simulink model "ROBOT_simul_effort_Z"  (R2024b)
settings: Solver=VariableStepAuto  StartTime=0.0  StopTime=5  RelTol=1e-3
undefined symbols (not defined in the file): a, ARRIERE_Defaut_sldprt, avant01_Defaut_sldprt, avant02_Defaut_sldprt, avant03_Defaut_sldprt, avant1_Defaut_sldprt, AXE, BASE_Defaut_sldprt, BIELLE, BIELLE_Defaut_sldprt, BRAS_Defaut_sldprt, bras_Defaut_sldprt, C_Realiste_sldprt, CABLE_Defaut_sldprt, cable_Defaut_sldprt, CACHE_Defaut_sldprt, CARTE, carte_Defaut_sldprt, CARTER, carter, CHC, CODEUR_Defaut_sldprt, cruciforme, cylindrique, deg, Drive, Fichiers, Fichiers_Matlab_sujetA, FIXATION, fixation_Defaut_sldprt, H, HEXAGONALE_Defaut_sldprt, joint_Defaut_sldprt, kg, m, M4, M4_Defaut_sldprt, manette1_Defaut_sldprt, manette2_Defaut_sldprt, MATLAB, Matlab, matlab_Defaut_sldprt, mm, modif, MOTEUR_Defaut_sldprt, N, NEZ_Defaut_sldprt, nom, palier, PARALLELOGRAMME_Defaut_sldprt, petite, plaque, rad, Ressort, Rondelle, ROTOR_Defaut_sldprt, s, SET, simple, socle_Defaut_sldprt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
libraries: sm_lib x463, fl_lib x45, nesl_utility x27, simulink x2
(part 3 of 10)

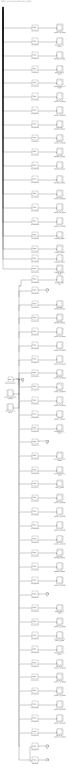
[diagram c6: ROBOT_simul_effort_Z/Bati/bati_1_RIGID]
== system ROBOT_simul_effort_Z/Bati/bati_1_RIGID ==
  CACHE_1_RIGID : Subsystem
  CACHE_2_RIGID : Subsystem
  CACHE_3_RIGID : Subsystem
  CARTER_ARRIERE_1_RIGID : Subsystem
  CARTE_HEXAGONALE_1_RIGID : Subsystem
  FIXATION_MOTEUR_1_RIGID : Subsystem
  FIXATION_MOTEUR_2_RIGID : Subsystem
  FIXATION_MOTEUR_3_RIGID : Subsystem
  FIXATION_MOTEUR_4_RIGID : Subsystem
  FIXATION_MOTEUR_5_RIGID : Subsystem
  FIXATION_MOTEUR_6_RIGID : Subsystem
  MOTEUR_1_RIGID : Subsystem
  MOTEUR_2_RIGID : Subsystem
  MOTEUR_3_RIGID : Subsystem
  PLAQUE_NOM_1_RIGID : Subsystem
  PLAQUE_NOM_SET : Subsystem
  ReferenceFrame : sm_lib/Frames and Transforms/Reference Frame
  Rondelle_M4_1_RIGID : Subsystem
  Rondelle_M4_2_RIGID : Subsystem
  Transform : sm_lib/Frames and Transforms/Rigid Transform  RotationMethod=ArbitraryAxis  FollAlignAxisA=+X  BaseAlignAxisA=+Y  FollAlignAxisB=+Y  BaseAlignAxisB=+Z  RotationStandardAxis=+Z  RotationAngle=2.2576709855630241  RotationAngleUnits=rad  RotationArbitraryAxis=[-0.47317816576134769 -0.62293756647304832 0.62293756647304788]  RotationSequenceAxes=FollowerAxes  RotationSequence=XYX  RotationSequenceAngles=[0 0 0]  RotationSequenceAnglesUnits=deg  RotationMatrix=[1 0 0; 0 1 0; 0 0 1]  Quaternion=[1 0 0 0]  TranslationMethod=Cartesian  TranslationCartesianOffset=[-67.982453021745741 154.13917308955064 38.499999999999979]  TranslationCartesianOffsetUnits=mm  TranslationStandardAxis=+Z  TranslationStandardOffset=0  TranslationStandardOffsetUnits=mm  TranslationROffset=0  TranslationROffsetUnits=m  TranslationThetaOffset=0  TranslationThetaOffsetUnits=deg  TranslationZOffset=0  TranslationZOffsetUnits=m
  Transform1 : sm_lib/Frames and Transforms/Rigid Transform  RotationMethod=ArbitraryAxis  FollAlignAxisA=+X  BaseAlignAxisA=+Y  FollAlignAxisB=+Y  BaseAlignAxisB=+Z  RotationStandardAxis=+Z  RotationAngle=2.2455218567975841  RotationAngleUnits=rad  RotationArbitraryAxis=[-0.62007686508407689 -0.48063433374552811 -0.62007686508407622]  RotationSequenceAxes=FollowerAxes  RotationSequence=XYX  RotationSequenceAngles=[0 0 0]  RotationSequenceAnglesUnits=deg  RotationMatrix=[1 0 0; 0 1 0; 0 0 1]  Quaternion=[1 0 0 0]  TranslationMethod=Cartesian  TranslationCartesianOffset=[67.670238338594061 154.67994478363838 38.499999999999979]  TranslationCartesianOffsetUnits=mm  TranslationStandardAxis=+Z  TranslationStandardOffset=0  TranslationStandardOffsetUnits=mm  TranslationROffset=0  TranslationROffsetUnits=m  TranslationThetaOffset=0  TranslationThetaOffsetUnits=deg  TranslationZOffset=0  TranslationZOffsetUnits=m
  Transform10 : sm_lib/Frames and Transforms/Rigid Transform  RotationMethod=ArbitraryAxis  FollAlignAxisA=+X  BaseAlignAxisA=+Y  FollAlignAxisB=+Y  BaseAlignAxisB=+Z  RotationStandardAxis=+Z  RotationAngle=1.5874169403231204  RotationAngleUnits=rad  RotationArbitraryAxis=[0.12785986324311854 -0.98351599414696989 0.12785986324311688]  RotationSequenceAxes=FollowerAxes  RotationSequence=XYX  RotationSequenceAngles=[0 0 0]  RotationSequenceAnglesUnits=deg  RotationMatrix=[1 0 0; 0 1 0; 0 0 1]  Quaternion=[1 0 0 0]  TranslationMethod=Cartesian  TranslationCartesianOffset=[-21.302011487444762 191.53150356202462 36.100000000000051]  TranslationCartesianOffsetUnits=mm  TranslationStandardAxis=+Z  TranslationStandardOffset=0  TranslationStandardOffsetUnits=mm  TranslationROffset=0  TranslationROffsetUnits=m  TranslationThetaOffset=0  TranslationThetaOffsetUnits=deg  TranslationZOffset=0  TranslationZOffsetUnits=m
  Transform11 : sm_lib/Frames and Transforms/Rigid Transform  RotationMethod=ArbitraryAxis  FollAlignAxisA=+X  BaseAlignAxisA=+Y  FollAlignAxisB=+Y  BaseAlignAxisB=+Z  RotationStandardAxis=+Z  RotationAngle=2.557922199918194  RotationAngleUnits=rad  RotationArbitraryAxis=[0.67444507075713422 -0.30041253812517366 0.67444507075713389]  RotationSequenceAxes=FollowerAxes  RotationSequence=XYX  RotationSequenceAngles=[0 0 0]  RotationSequenceAnglesUnits=deg  RotationMatrix=[1 0 0; 0 1 0; 0 0 1]  Quaternion=[1 0 0 0]  TranslationMethod=Cartesian  TranslationCartesianOffset=[-8.6943864691458312 146.25405010671241 36.099999999999994]  TranslationCartesianOffsetUnits=mm  TranslationStandardAxis=+Z  TranslationStandardOffset=0  TranslationStandardOffsetUnits=mm  TranslationROffset=0  TranslationROffsetUnits=m  TranslationThetaOffset=0  TranslationThetaOffsetUnits=deg  TranslationZOffset=0  TranslationZOffsetUnits=m
  Transform12 : sm_lib/Frames and Transforms/Rigid Transform  RotationMethod=ArbitraryAxis  FollAlignAxisA=+X  BaseAlignAxisA=+Y  FollAlignAxisB=+Y  BaseAlignAxisB=+Z  RotationStandardAxis=+Z  RotationAngle=1.5816892610060764  RotationAngleUnits=rad  RotationArbitraryAxis=[0.10380436397422958 -0.98916596587216399 0.10380436397423064]  RotationSequenceAxes=FollowerAxes  RotationSequence=XYX  RotationSequenceAngles=[0 0 0]  RotationSequenceAnglesUnits=deg  RotationMatrix=[1 0 0; 0 1 0; 0 0 1]  Quaternion=[1 0 0 0]  TranslationMethod=Cartesian  TranslationCartesianOffset=[31.197488247191473 107.27753449924363 36.099999999999994]  TranslationCartesianOffsetUnits=mm  TranslationStandardAxis=+Z  TranslationStandardOffset=0  TranslationStandardOffsetUnits=mm  TranslationROffset=0  TranslationROffsetUnits=m  TranslationThetaOffset=0  TranslationThetaOffsetUnits=deg  TranslationZOffset=0  TranslationZOffsetUnits=m
  Transform13 : sm_lib/Frames and Transforms/Rigid Transform  RotationMethod=ArbitraryAxis  FollAlignAxisA=+X  BaseAlignAxisA=+Y  FollAlignAxisB=+Y  BaseAlignAxisB=+Z  RotationStandardAxis=+Z  RotationAngle=2.4188584057763718  RotationAngleUnits=rad  RotationArbitraryAxis=[-0.65465367070797598 -0.37796447300923064 -0.6546536707079762]  RotationSequenceAxes=FollowerAxes  RotationSequence=XYX  RotationSequenceAngles=[0 0 0]  RotationSequenceAnglesUnits=deg  RotationMatrix=[1 0 0; 0 1 0; 0 0 1]  Quaternion=[1 0 0 0]  TranslationMethod=Cartesian  TranslationCartesianOffset=[-32.1104315373926 141.51053427005223 49.100000000000001]  TranslationCartesianOffsetUnits=mm  TranslationStandardAxis=+Z  TranslationStandardOffset=0  TranslationStandardOffsetUnits=mm  TranslationROffset=0  TranslationROffsetUnits=m  TranslationThetaOffset=0  TranslationThetaOffsetUnits=deg  TranslationZOffset=0  TranslationZOffsetUnits=m
  Transform14 : sm_lib/Frames and Transforms/Rigid Transform  RotationMethod=ArbitraryAxis  FollAlignAxisA=+X  BaseAlignAxisA=+Y  FollAlignAxisB=+Y  BaseAlignAxisB=+Z  RotationStandardAxis=+Z  RotationAngle=2.253606277940353  RotationAngleUnits=rad  RotationArbitraryAxis=[-0.62198874395633519 -0.47566795643940651 -0.62198874395633508]  RotationSequenceAxes=FollowerAxes  RotationSequence=XYX  RotationSequenceAngles=[0 0 0]  RotationSequenceAnglesUnits=deg  RotationMatrix=[1 0 0; 0 1 0; 0 0 1]  Quaternion=[1 0 0 0]  TranslationMethod=Cartesian  TranslationCartesianOffset=[76.71272566730876 95.557331318822435 36.100000000000051]  TranslationCartesianOffsetUnits=mm  TranslationStandardAxis=+Z  TranslationStandardOffset=0  TranslationStandardOffsetUnits=mm  TranslationROffset=0  TranslationROffsetUnits=m  TranslationThetaOffset=0  TranslationThetaOffsetUnits=deg  TranslationZOffset=0  TranslationZOffsetUnits=m
  Transform15 : sm_lib/Frames and Transforms/Rigid Transform  RotationMethod=ArbitraryAxis  FollAlignAxisA=+X  BaseAlignAxisA=+Y  FollAlignAxisB=+Y  BaseAlignAxisB=+Z  RotationStandardAxis=+Z  RotationAngle=2.1395291955010958  RotationAngleUnits=rad  RotationArbitraryAxis=[-0.59164485304725056 -0.54764289069191197 -0.59164485304725156]  RotationSequenceAxes=FollowerAxes  RotationSequence=XYX  RotationSequenceAngles=[0 0 0]  RotationSequenceAnglesUnits=deg  RotationMatrix=[1 0 0; 0 1 0; 0 0 1]  Quaternion=[1 0 0 0]  TranslationMethod=Cartesian  TranslationCartesianOffset=[39.05251803832482 137.78242766379034 36.099999999999966]  TranslationCartesianOffsetUnits=mm  TranslationStandardAxis=+Z  TranslationStandardOffset=0  TranslationStandardOffsetUnits=mm  TranslationROffset=0  TranslationROffsetUnits=m  TranslationThetaOffset=0  TranslationThetaOffsetUnits=deg  TranslationZOffset=0  TranslationZOffsetUnits=m
  Transform16 : sm_lib/Frames and Transforms/Rigid Transform  RotationMethod=ArbitraryAxis  FollAlignAxisA=+X  BaseAlignAxisA=+Y  FollAlignAxisB=+Y  BaseAlignAxisB=+Z  RotationStandardAxis=+Z  RotationAngle=0.1305039651717789  RotationAngleUnits=rad  RotationArbitraryAxis=[1.6038157489539324e-15 1 -1.2797090690177757e-15]  RotationSequenceAxes=FollowerAxes  RotationSequence=XYX  RotationSequenceAngles=[0 0 0]  RotationSequenceAnglesUnits=deg  RotationMatrix=[1 0 0; 0 1 0; 0 0 1]  Quaternion=[1 0 0 0]  TranslationMethod=Cartesian  TranslationCartesianOffset=[-9.8750000000000053 1.2000000000000066 14.050000000000008]  TranslationCartesianOffsetUnits=mm  TranslationStandardAxis=+Z  TranslationStandardOffset=0  TranslationStandardOffsetUnits=mm  TranslationROffset=0  TranslationROffsetUnits=m  TranslationThetaOffset=0  TranslationThetaOffsetUnits=deg  TranslationZOffset=0  TranslationZOffsetUnits=m
  Transform17 : sm_lib/Frames and Transforms/Rigid Transform  RotationMethod=ArbitraryAxis  FollAlignAxisA=+X  BaseAlignAxisA=+Y  FollAlignAxisB=+Y  BaseAlignAxisB=+Z  RotationStandardAxis=+Z  RotationAngle=3.1415926535897931  RotationAngleUnits=rad  RotationArbitraryAxis=[-0.14780941112961105 0.98901586336191671 0]  RotationSequenceAxes=FollowerAxes  RotationSequence=XYX  RotationSequenceAngles=[0 0 0]  RotationSequenceAnglesUnits=deg  RotationMatrix=[1 0 0; 0 1 0; 0 0 1]  Quaternion=[1 0 0 0]  TranslationMethod=Cartesian  TranslationCartesianOffset=[0 115.25000000000001 16.899999999999999]  TranslationCartesianOffsetUnits=mm  TranslationStandardAxis=+Z  TranslationStandardOffset=0  TranslationStandardOffsetUnits=mm  TranslationROffset=0  TranslationROffsetUnits=m  TranslationThetaOffset=0  TranslationThetaOffsetUnits=deg  TranslationZOffset=0  TranslationZOffsetUnits=m
  Transform18 : sm_lib/Frames and Transforms/Rigid Transform  RotationMethod=ArbitraryAxis  FollAlignAxisA=+X  BaseAlignAxisA=+Y  FollAlignAxisB=+Y  BaseAlignAxisB=+Z  RotationStandardAxis=+Z  RotationAngle=3.1415926535897909  RotationAngleUnits=rad  RotationArbitraryAxis=[-0.70710678118654757 -1.2168216554799258e-15 -0.70710678118654746]  RotationSequenceAxes=FollowerAxes  RotationSequence=XYX  RotationSequenceAngles=[0 0 0]  RotationSequenceAnglesUnits=deg  RotationMatrix=[1 0 0; 0 1 0; 0 0 1]  Quaternion=[1 0 0 0]  TranslationMethod=Cartesian  TranslationCartesianOffset=[0 115.25000000000001 -1.799999999999996]  TranslationCartesianOffsetUnits=mm  TranslationStandardAxis=+Z  TranslationStandardOffset=0  TranslationStandardOffsetUnits=mm  TranslationROffset=0  TranslationROffsetUnits=m  TranslationThetaOffset=0  TranslationThetaOffsetUnits=deg  TranslationZOffset=0  TranslationZOffsetUnits=m
  Transform19 : sm_lib/Frames and Transforms/Rigid Transform  RotationMethod=ArbitraryAxis  FollAlignAxisA=+X  BaseAlignAxisA=+Y  FollAlignAxisB=+Y  BaseAlignAxisB=+Z  RotationStandardAxis=+Z  RotationAngle=3.1415926535897931  RotationAngleUnits=rad  RotationArbitraryAxis=[-0.62251463663761875 0.78260815685241447 9.5278235956943858e-17]  RotationSequenceAxes=FollowerAxes  RotationSequence=XYX  RotationSequenceAngles=[0 0 0]  RotationSequenceAnglesUnits=deg  RotationMatrix=[1 0 0; 0 1 0; 0 0 1]  Quaternion=[1 0 0 0]  TranslationMethod=Cartesian  TranslationCartesianOffset=[-5.4923264138695282 106.15877278095202 52.900000000000013]  TranslationCartesianOffsetUnits=mm  TranslationStandardAxis=+Z  TranslationStandardOffset=0  TranslationStandardOffsetUnits=mm  TranslationROffset=0  TranslationROffsetUnits=m  TranslationThetaOffset=0  TranslationThetaOffsetUnits=deg  TranslationZOffset=0  TranslationZOffsetUnits=m
  Transform2 : sm_lib/Frames and Transforms/Rigid Transform  RotationMethod=ArbitraryAxis  FollAlignAxisA=+X  BaseAlignAxisA=+Y  FollAlignAxisB=+Y  BaseAlignAxisB=+Z  RotationStandardAxis=+Z  RotationAngle=1.7212826903554606  RotationAngleUnits=rad  RotationArbitraryAxis=[0.85979818153437826 0.36107276761767659 0.36107276761767548]  RotationSequenceAxes=FollowerAxes  RotationSequence=XYX  RotationSequenceAngles=[0 0 0]  RotationSequenceAnglesUnits=deg  RotationMatrix=[1 0 0; 0 1 0; 0 0 1]  Quaternion=[1 0 0 0]  TranslationMethod=Cartesian  TranslationCartesianOffset=[0.3122146831511497 36.930882126810701 38.499999999999979]  TranslationCartesianOffsetUnits=mm  TranslationStandardAxis=+Z  TranslationStandardOffset=0  TranslationStandardOffsetUnits=mm  TranslationROffset=0  TranslationROffsetUnits=m  TranslationThetaOffset=0  TranslationThetaOffsetUnits=deg  TranslationZOffset=0  TranslationZOffsetUnits=m
  Transform20 : sm_lib/Frames and Transforms/Rigid Transform  RotationMethod=ArbitraryAxis  FollAlignAxisA=+X  BaseAlignAxisA=+Y  FollAlignAxisB=+Y  BaseAlignAxisB=+Z  RotationStandardAxis=+Z  RotationAngle=1.5707963267948968  RotationAngleUnits=rad  RotationArbitraryAxis=[-0 -1 -1.8723979605913744e-16]  RotationSequenceAxes=FollowerAxes  RotationSequence=XYX  RotationSequenceAngles=[0 0 0]  RotationSequenceAnglesUnits=deg  RotationMatrix=[1 0 0; 0 1 0; 0 0 1]  Quaternion=[1 0 0 0]  TranslationMethod=Cartesian  TranslationCartesianOffset=[-6.6870740261211532 74.311283427110965 49.100000000000001]  TranslationCartesianOffsetUnits=mm  TranslationStandardAxis=+Z  TranslationStandardOffset=0  TranslationStandardOffsetUnits=mm  TranslationROffset=0  TranslationROffsetUnits=m  TranslationThetaOffset=0  TranslationThetaOffsetUnits=deg  TranslationZOffset=0  TranslationZOffsetUnits=m
  Transform21 : sm_lib/Frames and Transforms/Rigid Transform  RotationMethod=ArbitraryAxis  FollAlignAxisA=+X  BaseAlignAxisA=+Y  FollAlignAxisB=+Y  BaseAlignAxisB=+Z  RotationStandardAxis=+Z  RotationAngle=2.5869353710023297  RotationAngleUnits=rad  RotationArbitraryAxis=[-0.28466429222446077 0.67785184248932562 -0.6778518424893254]  RotationSequenceAxes=FollowerAxes  RotationSequence=XYX  RotationSequenceAngles=[0 0 0]  RotationSequenceAnglesUnits=deg  RotationMatrix=[1 0 0; 0 1 0; 0 0 1]  Quaternion=[1 0 0 0]  TranslationMethod=Cartesian  TranslationCartesianOffset=[-16.466410454294302 53.38468832772007 38.500000000000007]  TranslationCartesianOffsetUnits=mm  TranslationStandardAxis=+Z  TranslationStandardOffset=0  TranslationStandardOffsetUnits=mm  TranslationROffset=0  TranslationROffsetUnits=m  TranslationThetaOffset=0  TranslationThetaOffsetUnits=deg  TranslationZOffset=0  TranslationZOffsetUnits=m
  Transform22 : sm_lib/Frames and Transforms/Rigid Transform  RotationMethod=ArbitraryAxis  FollAlignAxisA=+X  BaseAlignAxisA=+Y  FollAlignAxisB=+Y  BaseAlignAxisB=+Z  RotationStandardAxis=+Z  RotationAngle=2.5869353710023297  RotationAngleUnits=rad  RotationArbitraryAxis=[-0.28466429222446077 0.67785184248932562 -0.67785184248932528]  RotationSequenceAxes=FollowerAxes  RotationSequence=XYX  RotationSequenceAngles=[0 0 0]  RotationSequenceAnglesUnits=deg  RotationMatrix=[1 0 0; 0 1 0; 0 0 1]  Quaternion=[1 0 0 0]  TranslationMethod=Cartesian  TranslationCartesianOffset=[-38.956907978955229 75.439790256598585 38.500000000000028]  TranslationCartesianOffsetUnits=mm  TranslationStandardAxis=+Z  TranslationStandardOffset=0  TranslationStandardOffsetUnits=mm  TranslationROffset=0  TranslationROffsetUnits=m  TranslationThetaOffset=0  TranslationThetaOffsetUnits=deg  TranslationZOffset=0  TranslationZOffsetUnits=m
  Transform23 : sm_lib/Frames and Transforms/Rigid Transform  RotationMethod=ArbitraryAxis  FollAlignAxisA=+X  BaseAlignAxisA=+Y  FollAlignAxisB=+Y  BaseAlignAxisB=+Z  RotationStandardAxis=+Z  RotationAngle=2.1079572963404796  RotationAngleUnits=rad  RotationArbitraryAxis=[0.58180115951651357 -0.56834392894662011 0.58180115951651357]  RotationSequenceAxes=FollowerAxes  RotationSequence=XYX  RotationSequenceAngles=[0 0 0]  RotationSequenceAnglesUnits=deg  RotationMatrix=[1 0 0; 0 1 0; 0 0 1]  Quaternion=[1 0 0 0]  TranslationMethod=Cartesian  TranslationCartesianOffset=[-32.920216655203667 36.606063190274597 36.100000000000037]  TranslationCartesianOffsetUnits=mm  TranslationStandardAxis=+Z  TranslationStandardOffset=0  TranslationStandardOffsetUnits=mm  TranslationROffset=0  TranslationROffsetUnits=m  TranslationThetaOffset=0  TranslationThetaOffsetUnits=deg  TranslationZOffset=0  TranslationZOffsetUnits=m
  Transform24 : sm_lib/Frames and Transforms/Rigid Transform  RotationMethod=ArbitraryAxis  FollAlignAxisA=+X  BaseAlignAxisA=+Y  FollAlignAxisB=+Y  BaseAlignAxisB=+Z  RotationStandardAxis=+Z  RotationAngle=2.5913633997650876  RotationAngleUnits=rad  RotationArbitraryAxis=[0.67835179231251819 -0.28227237153641171 0.67835179231251697]  RotationSequenceAxes=FollowerAxes  RotationSequence=XYX  RotationSequenceAngles=[0 0 0]  RotationSequenceAnglesUnits=deg  RotationMatrix=[1 0 0; 0 1 0; 0 0 1]  Quaternion=[1 0 0 0]  TranslationMethod=Cartesian  TranslationCartesianOffset=[-55.410714179864605 58.661165119153118 36.100000000000051]  TranslationCartesianOffsetUnits=mm  TranslationStandardAxis=+Z  TranslationStandardOffset=0  TranslationStandardOffsetUnits=mm  TranslationROffset=0  TranslationROffsetUnits=m  TranslationThetaOffset=0  TranslationThetaOffsetUnits=deg  TranslationZOffset=0  TranslationZOffsetUnits=m
  Transform25 : sm_lib/Frames and Transforms/Rigid Transform  RotationMethod=ArbitraryAxis  FollAlignAxisA=+X  BaseAlignAxisA=+Y  FollAlignAxisB=+Y  BaseAlignAxisB=+Z  RotationStandardAxis=+Z  RotationAngle=2.7200049334585095  RotationAngleUnits=rad  RotationArbitraryAxis=[0.6907299635194234 -0.21397250990001554 0.6907299635194234]  RotationSequenceAxes=FollowerAxes  RotationSequence=XYX  RotationSequenceAngles=[0 0 0]  RotationSequenceAnglesUnits=deg  RotationMatrix=[1 0 0; 0 1 0; 0 0 1]  Quaternion=[1 0 0 0]  TranslationMethod=Cartesian  TranslationCartesianOffset=[-0.012604253384927124 70.163313465165515 36.099999999999966]  TranslationCartesianOffsetUnits=mm  TranslationStandardAxis=+Z  TranslationStandardOffset=0  TranslationStandardOffsetUnits=mm  TranslationROffset=0  TranslationROffsetUnits=m  TranslationThetaOffset=0  TranslationThetaOffsetUnits=deg  TranslationZOffset=0  TranslationZOffsetUnits=m
  Transform26 : sm_lib/Frames and Transforms/Rigid Transform  RotationMethod=ArbitraryAxis  FollAlignAxisA=+X  BaseAlignAxisA=+Y  FollAlignAxisB=+Y  BaseAlignAxisB=+Z  RotationStandardAxis=+Z  RotationAngle=2.2845314039372839  RotationAngleUnits=rad  RotationArbitraryAxis=[-0.62900467206978528 -0.4568437862429186 -0.62900467206978417]  RotationSequenceAxes=FollowerAxes  RotationSequence=XYX  RotationSequenceAngles=[0 0 0]  RotationSequenceAnglesUnits=deg  RotationMatrix=[1 0 0; 0 1 0; 0 0 1]  Quaternion=[1 0 0 0]  TranslationMethod=Cartesian  TranslationCartesianOffset=[-22.503101778045874 92.21841539404403 36.099999999999994]  TranslationCartesianOffsetUnits=mm  TranslationStandardAxis=+Z  TranslationStandardOffset=0  TranslationStandardOffsetUnits=mm  TranslationROffset=0  TranslationROffsetUnits=m  TranslationThetaOffset=0  TranslationThetaOffsetUnits=deg  TranslationZOffset=0  TranslationZOffsetUnits=m
  Transform27 : sm_lib/Frames and Transforms/Rigid Transform  RotationMethod=ArbitraryAxis  FollAlignAxisA=+X  BaseAlignAxisA=+Y  FollAlignAxisB=+Y  BaseAlignAxisB=+Z  RotationStandardAxis=+Z  RotationAngle=1.5707963267948961  RotationAngleUnits=rad  RotationArbitraryAxis=[-1 0 0]  RotationSequenceAxes=FollowerAxes  RotationSequence=XYX  RotationSequenceAngles=[0 0 0]  RotationSequenceAnglesUnits=deg  RotationMatrix=[1 0 0; 0 1 0; 0 0 1]  Quaternion=[1 0 0 0]  TranslationMethod=Cartesian  TranslationCartesianOffset=[0 -1.5000000000000151 37.700000000000003]  TranslationCartesianOffsetUnits=mm  TranslationStandardAxis=+Z  TranslationStandardOffset=0  TranslationStandardOffsetUnits=mm  TranslationROffset=0  TranslationROffsetUnits=m  TranslationThetaOffset=0  TranslationThetaOffsetUnits=deg  TranslationZOffset=0  TranslationZOffsetUnits=m
  Transform28 : sm_lib/Frames and Transforms/Rigid Transform  RotationMethod=ArbitraryAxis  FollAlignAxisA=+X  BaseAlignAxisA=+Y  FollAlignAxisB=+Y  BaseAlignAxisB=+Z  RotationStandardAxis=+Z  RotationAngle=2.773492570857111  RotationAngleUnits=rad  RotationArbitraryAxis=[0.18615678789738549 -0.69474659060686594 0.69474659060686572]  RotationSequenceAxes=FollowerAxes  RotationSequence=XYX  RotationSequenceAngles=[0 0 0]  RotationSequenceAnglesUnits=deg  RotationMatrix=[1 0 0; 0 1 0; 0 0 1]  Quaternion=[1 0 0 0]  TranslationMethod=Cartesian  TranslationCartesianOffset=[9.8750000000000089 31.199999999999992 14.050000000000008]  TranslationCartesianOffsetUnits=mm  TranslationStandardAxis=+Z  TranslationStandardOffset=0  TranslationStandardOffsetUnits=mm  TranslationROffset=0  TranslationROffsetUnits=m  TranslationThetaOffset=0  TranslationThetaOffsetUnits=deg  TranslationZOffset=0  TranslationZOffsetUnits=m
  Transform29 : sm_lib/Frames and Transforms/Rigid Transform  RotationMethod=ArbitraryAxis  FollAlignAxisA=+X  BaseAlignAxisA=+Y  FollAlignAxisB=+Y  BaseAlignAxisB=+Z  RotationStandardAxis=+Z  RotationAngle=2.773492570857111  RotationAngleUnits=rad  RotationArbitraryAxis=[0.18615678789738549 -0.69474659060686594 0.69474659060686572]  RotationSequenceAxes=FollowerAxes  RotationSequence=XYX  RotationSequenceAngles=[0 0 0]  RotationSequenceAnglesUnits=deg  RotationMatrix=[1 0 0; 0 1 0; 0 0 1]  Quaternion=[1 0 0 0]  TranslationMethod=Cartesian  TranslationCartesianOffset=[-9.8750000000000053 31.199999999999992 14.050000000000008]  TranslationCartesianOffsetUnits=mm  TranslationStandardAxis=+Z  TranslationStandardOffset=0  TranslationStandardOffsetUnits=mm  TranslationROffset=0  TranslationROffsetUnits=m  TranslationThetaOffset=0  TranslationThetaOffsetUnits=deg  TranslationZOffset=0  TranslationZOffsetUnits=m
  Transform3 : sm_lib/Frames and Transforms/Rigid Transform  RotationMethod=ArbitraryAxis  FollAlignAxisA=+X  BaseAlignAxisA=+Y  FollAlignAxisB=+Y  BaseAlignAxisB=+Z  RotationStandardAxis=+Z  RotationAngle=1.7212826903554632  RotationAngleUnits=rad  RotationArbitraryAxis=[0.85979818153438259 0.36107276761767909 0.36107276761766205]  RotationSequenceAxes=FollowerAxes  RotationSequence=XYX  RotationSequenceAngles=[0 0 0]  RotationSequenceAnglesUnits=deg  RotationMatrix=[1 0 0; 0 1 0; 0 0 1]  Quaternion=[1 0 0 0]  TranslationMethod=Cartesian  TranslationCartesianOffset=[-106.82639785458468 167.86430788780581 99.318100970001225]  TranslationCartesianOffsetUnits=mm  TranslationStandardAxis=+Z  TranslationStandardOffset=0  TranslationStandardOffsetUnits=mm  TranslationROffset=0  TranslationROffsetUnits=m  TranslationThetaOffset=0  TranslationThetaOffsetUnits=deg  TranslationZOffset=0  TranslationZOffsetUnits=m
  Transform30 : sm_lib/Frames and Transforms/Rigid Transform  RotationMethod=ArbitraryAxis  FollAlignAxisA=+X  BaseAlignAxisA=+Y  FollAlignAxisB=+Y  BaseAlignAxisB=+Z  RotationStandardAxis=+Z  RotationAngle=3.1415926535897931  RotationAngleUnits=rad  RotationArbitraryAxis=[-0.99787184465383982 -0 0.065205687230048659]  RotationSequenceAxes=FollowerAxes  RotationSequence=XYX  RotationSequenceAngles=[0 0 0]  RotationSequenceAnglesUnits=deg  RotationMatrix=[1 0 0; 0 1 0; 0 0 1]  Quaternion=[1 0 0 0]  TranslationMethod=Cartesian  TranslationCartesianOffset=[9.8750000000000089 2.0000000000000018 14.050000000000008]  TranslationCartesianOffsetUnits=mm  TranslationStandardAxis=+Z  TranslationStandardOffset=0  TranslationStandardOffsetUnits=mm  TranslationROffset=0  TranslationROffsetUnits=m  TranslationThetaOffset=0  TranslationThetaOffsetUnits=deg  TranslationZOffset=0  TranslationZOffsetUnits=m
  Transform31 : sm_lib/Frames and Transforms/Rigid Transform  RotationMethod=ArbitraryAxis  FollAlignAxisA=+X  BaseAlignAxisA=+Y  FollAlignAxisB=+Y  BaseAlignAxisB=+Z  RotationStandardAxis=+Z  RotationAngle=3.1415926535897931  RotationAngleUnits=rad  RotationArbitraryAxis=[0 1 0]  RotationSequenceAxes=FollowerAxes  RotationSequence=XYX  RotationSequenceAngles=[0 0 0]  RotationSequenceAnglesUnits=deg  RotationMatrix=[1 0 0; 0 1 0; 0 0 1]  Quaternion=[1 0 0 0]  TranslationMethod=None  TranslationCartesianOffset=[0 0 0]  TranslationCartesianOffsetUnits=m  TranslationStandardAxis=+Z  TranslationStandardOffset=0  TranslationStandardOffsetUnits=m  TranslationROffset=0  TranslationROffsetUnits=m  TranslationThetaOffset=0  TranslationThetaOffsetUnits=deg  TranslationZOffset=0  TranslationZOffsetUnits=m
  Transform32 : sm_lib/Frames and Transforms/Rigid Transform  RotationMethod=ArbitraryAxis  FollAlignAxisA=+X  BaseAlignAxisA=+Y  FollAlignAxisB=+Y  BaseAlignAxisB=+Z  RotationStandardAxis=+Z  RotationAngle=1.6591931073504684  RotationAngleUnits=rad  RotationArbitraryAxis=[-0.28481620059537222 -0.91529201010214944 -0.28481620059537222]  RotationSequenceAxes=FollowerAxes  RotationSequence=XYX  RotationSequenceAngles=[0 0 0]  RotationSequenceAnglesUnits=deg  RotationMatrix=[1 0 0; 0 1 0; 0 0 1]  Quaternion=[1 0 0 0]  TranslationMethod=Cartesian  TranslationCartesianOffset=[78.177113545509911 88.894999319852587 19.199999999999996]  TranslationCartesianOffsetUnits=mm  TranslationStandardAxis=+Z  TranslationStandardOffset=0  TranslationStandardOffsetUnits=mm  TranslationROffset=0  TranslationROffsetUnits=m  TranslationThetaOffset=0  TranslationThetaOffsetUnits=deg  TranslationZOffset=0  TranslationZOffsetUnits=m
  Transform33 : sm_lib/Frames and Transforms/Rigid Transform  RotationMethod=ArbitraryAxis  FollAlignAxisA=+X  BaseAlignAxisA=+Y  FollAlignAxisB=+Y  BaseAlignAxisB=+Z  RotationStandardAxis=+Z  RotationAngle=1.5707963267948968  RotationAngleUnits=rad  RotationArbitraryAxis=[-0 -1 -0]  RotationSequenceAxes=FollowerAxes  RotationSequence=XYX  RotationSequenceAngles=[0 0 0]  RotationSequenceAnglesUnits=deg  RotationMatrix=[1 0 0; 0 1 0; 0 0 1]  Quaternion=[1 0 0 0]  TranslationMethod=Cartesian  TranslationCartesianOffset=[56.590549141302901 55.218676943733961 19.199999999999996]  TranslationCartesianOffsetUnits=mm  TranslationStandardAxis=+Z  TranslationStandardOffset=0  TranslationStandardOffsetUnits=mm  TranslationROffset=0  TranslationROffsetUnits=m  TranslationThetaOffset=0  TranslationThetaOffsetUnits=deg  TranslationZOffset=0  TranslationZOffsetUnits=m
  Transform34 : sm_lib/Frames and Transforms/Rigid Transform  RotationMethod=ArbitraryAxis  FollAlignAxisA=+X  BaseAlignAxisA=+Y  FollAlignAxisB=+Y  BaseAlignAxisB=+Z  RotationStandardAxis=+Z  RotationAngle=2.4188584057763807  RotationAngleUnits=rad  RotationArbitraryAxis=[0.65465367070797764 -0.37796447300922553 0.65465367070797764]  RotationSequenceAxes=FollowerAxes  RotationSequence=XYX  RotationSequenceAngles=[0 0 0]  RotationSequenceAnglesUnits=deg  RotationMatrix=[1 0 0; 0 1 0; 0 0 1]  Quaternion=[1 0 0 0]  TranslationMethod=Cartesian  TranslationCartesianOffset=[23.693376218865065 194.27451469861313 19.199999999999996]  TranslationCartesianOffsetUnits=mm  TranslationStandardAxis=+Z  TranslationStandardOffset=0  TranslationStandardOffsetUnits=mm  TranslationROffset=0  TranslationROffsetUnits=m  TranslationThetaOffset=0  TranslationThetaOffsetUnits=deg  TranslationZOffset=0  TranslationZOffsetUnits=m
  Transform35 : sm_lib/Frames and Transforms/Rigid Transform  RotationMethod=ArbitraryAxis  FollAlignAxisA=+X  BaseAlignAxisA=+Y  FollAlignAxisB=+Y  BaseAlignAxisB=+Z  RotationStandardAxis=+Z  RotationAngle=2.4188584057763718  RotationAngleUnits=rad  RotationArbitraryAxis=[-0.65465367070797598 -0.37796447300923064 -0.65465367070797609]  RotationSequenceAxes=FollowerAxes  RotationSequence=XYX  RotationSequenceAngles=[0 0 0]  RotationSequenceAnglesUnits=deg  RotationMatrix=[1 0 0; 0 1 0; 0 0 1]  Quaternion=[1 0 0 0]  TranslationMethod=Cartesian  TranslationCartesianOffset=[-80.283925360168155 96.256808357652318 19.199999999999996]  TranslationCartesianOffsetUnits=mm  TranslationStandardAxis=+Z  TranslationStandardOffset=0  TranslationStandardOffsetUnits=mm  TranslationROffset=0  TranslationROffsetUnits=m  TranslationThetaOffset=0  TranslationThetaOffsetUnits=deg  TranslationZOffset=0  TranslationZOffsetUnits=m
  Transform36 : sm_lib/Frames and Transforms/Rigid Transform  RotationMethod=ArbitraryAxis  FollAlignAxisA=+X  BaseAlignAxisA=+Y  FollAlignAxisB=+Y  BaseAlignAxisB=+Z  RotationStandardAxis=+Z  RotationAngle=2.0489764020053052  RotationAngleUnits=rad  RotationArbitraryAxis=[0.56137820698022478 -0.60803701980663627 0.56137820698022478]  RotationSequenceAxes=FollowerAxes  RotationSequence=XYX  RotationSequenceAngles=[0 0 0]  RotationSequenceAnglesUnits=deg  RotationMatrix=[1 0 0; 0 1 0; 0 0 1]  Quaternion=[1 0 0 0]  TranslationMethod=Cartesian  TranslationCartesianOffset=[-16.264456666991514 196.13086666502576 19.199999999999996]  TranslationCartesianOffsetUnits=mm  TranslationStandardAxis=+Z  TranslationStandardOffset=0  TranslationStandardOffsetUnits=mm  TranslationROffset=0  TranslationROffsetUnits=m  TranslationThetaOffset=0  TranslationThetaOffsetUnits=deg  TranslationZOffset=0  TranslationZOffsetUnits=m
  Transform37 : sm_lib/Frames and Transforms/Rigid Transform  RotationMethod=ArbitraryAxis  FollAlignAxisA=+X  BaseAlignAxisA=+Y  FollAlignAxisB=+Y  BaseAlignAxisB=+Z  RotationStandardAxis=+Z  RotationAngle=2.8290477720117608  RotationAngleUnits=rad  RotationArbitraryAxis=[-0.69827493103712956 -0.15755710510854135 -0.69827493103712956]  RotationSequenceAxes=FollowerAxes  RotationSequence=XYX  RotationSequenceAngles=[0 0 0]  RotationSequenceAnglesUnits=deg  RotationMatrix=[1 0 0; 0 1 0; 0 0 1]  Quaternion=[1 0 0 0]  TranslationMethod=Cartesian  TranslationCartesianOffset=[-61.912656878518263 60.724134015121031 19.199999999999996]  TranslationCartesianOffsetUnits=mm  TranslationStandardAxis=+Z  TranslationStandardOffset=0  TranslationStandardOffsetUnits=mm  TranslationROffset=0  TranslationROffsetUnits=m  TranslationThetaOffset=0  TranslationThetaOffsetUnits=deg  TranslationZOffset=0  TranslationZOffsetUnits=m
  Transform38 : sm_lib/Frames and Transforms/Rigid Transform  RotationMethod=ArbitraryAxis  FollAlignAxisA=+X  BaseAlignAxisA=+Y  FollAlignAxisB=+Y  BaseAlignAxisB=+Z  RotationStandardAxis=+Z  RotationAngle=1.5865923302678127  RotationAngleUnits=rad  RotationArbitraryAxis=[-0.98432745245712761 0.12469856923650155 -0.1246985692365027]  RotationSequenceAxes=FollowerAxes  RotationSequence=XYX  RotationSequenceAngles=[0 0 0]  RotationSequenceAnglesUnits=deg  RotationMatrix=[1 0 0; 0 1 0; 0 0 1]  Quaternion=[1 0 0 0]  TranslationMethod=Cartesian  TranslationCartesianOffset=[61.810136748383464 131.92232607357974 38.500000000000007]  TranslationCartesianOffsetUnits=mm  TranslationStandardAxis=+Z  TranslationStandardOffset=0  TranslationStandardOffsetUnits=mm  TranslationROffset=0  TranslationROffsetUnits=m  TranslationThetaOffset=0  TranslationThetaOffsetUnits=deg  TranslationZOffset=0  TranslationZOffsetUnits=m
  Transform39 : sm_lib/Frames and Transforms/Rigid Transform  RotationMethod=ArbitraryAxis  FollAlignAxisA=+X  BaseAlignAxisA=+Y  FollAlignAxisB=+Y  BaseAlignAxisB=+Z  RotationStandardAxis=+Z  RotationAngle=2.2576709855630233  RotationAngleUnits=rad  RotationArbitraryAxis=[-0.47317816576134747 -0.62293756647304876 0.62293756647304765]  RotationSequenceAxes=FollowerAxes  RotationSequence=XYX  RotationSequenceAngles=[0 0 0]  RotationSequenceAnglesUnits=deg  RotationMatrix=[1 0 0; 0 1 0; 0 0 1]  Quaternion=[1 0 0 0]  TranslationMethod=Cartesian  TranslationCartesianOffset=[-45.343726294089642 160.44298559870006 38.500000000000007]  TranslationCartesianOffsetUnits=mm  TranslationStandardAxis=+Z  TranslationStandardOffset=0  TranslationStandardOffsetUnits=mm  TranslationROffset=0  TranslationROffsetUnits=m  TranslationThetaOffset=0  TranslationThetaOffsetUnits=deg  TranslationZOffset=0  TranslationZOffsetUnits=m
  Transform4 : sm_lib/Frames and Transforms/Rigid Transform  RotationMethod=ArbitraryAxis  FollAlignAxisA=+X  BaseAlignAxisA=+Y  FollAlignAxisB=+Y  BaseAlignAxisB=+Z  RotationStandardAxis=+Z  RotationAngle=2.2455218567975974  RotationAngleUnits=rad  RotationArbitraryAxis=[-0.62007686508408166 -0.48063433374552633 -0.62007686508407289]  RotationSequenceAxes=FollowerAxes  RotationSequence=XYX  RotationSequenceAngles=[0 0 0]  RotationSequenceAnglesUnits=deg  RotationMatrix=[1 0 0; 0 1 0; 0 0 1]  Quaternion=[1 0 0 0]  TranslationMethod=Cartesian  TranslationCartesianOffset=[7.8478716939170852 -3.5715282807566169 99.318100970001225]  TranslationCartesianOffsetUnits=mm  TranslationStandardAxis=+Z  TranslationStandardOffset=0  TranslationStandardOffsetUnits=mm  TranslationROffset=0  TranslationROffsetUnits=m  TranslationThetaOffset=0  TranslationThetaOffsetUnits=deg  TranslationZOffset=0  TranslationZOffsetUnits=m
  Transform40 : sm_lib/Frames and Transforms/Rigid Transform  RotationMethod=None  FollAlignAxisA=+X  BaseAlignAxisA=+Y  FollAlignAxisB=+Y  BaseAlignAxisB=+Z  RotationStandardAxis=+Z  RotationAngle=2.0835623886098844e-12  RotationAngleUnits=rad  RotationArbitraryAxis=[1 0 0]  RotationSequenceAxes=FollowerAxes  RotationSequence=XYX  RotationSequenceAngles=[0 0 0]  RotationSequenceAnglesUnits=deg  RotationMatrix=[1 0 0; 0 1 0; 0 0 1]  Quaternion=[1 0 0 0]  TranslationMethod=Cartesian  TranslationCartesianOffset=[-30 40 75]  TranslationCartesianOffsetUnits=mm  TranslationStandardAxis=+Z  TranslationStandardOffset=0  TranslationStandardOffsetUnits=mm  TranslationROffset=0  TranslationROffsetUnits=m  TranslationThetaOffset=0  TranslationThetaOffsetUnits=deg  TranslationZOffset=0  TranslationZOffsetUnits=m
  Transform41 : sm_lib/Frames and Transforms/Rigid Transform  RotationMethod=ArbitraryAxis  FollAlignAxisA=+X  BaseAlignAxisA=+Y  FollAlignAxisB=+Y  BaseAlignAxisB=+Z  RotationStandardAxis=+Z  RotationAngle=1.1415336785562208e-11  RotationAngleUnits=rad  RotationArbitraryAxis=[0 0 -1]  RotationSequenceAxes=FollowerAxes  RotationSequence=XYX  RotationSequenceAngles=[0 0 0]  RotationSequenceAnglesUnits=deg  RotationMatrix=[1 0 0; 0 1 0; 0 0 1]  Quaternion=[1 0 0 0]  TranslationMethod=Cartesian  TranslationCartesianOffset=[-1.3156175645385466e-09 0 24.000000000062251]  TranslationCartesianOffsetUnits=mm  TranslationStandardAxis=+Z  TranslationStandardOffset=0  TranslationStandardOffsetUnits=mm  TranslationROffset=0  TranslationROffsetUnits=m  TranslationThetaOffset=0  TranslationThetaOffsetUnits=deg  TranslationZOffset=0  TranslationZOffsetUnits=m
  Transform42 : sm_lib/Frames and Transforms/Rigid Transform  RotationMethod=ArbitraryAxis  FollAlignAxisA=+X  BaseAlignAxisA=+Y  FollAlignAxisB=+Y  BaseAlignAxisB=+Z  RotationStandardAxis=+Z  RotationAngle=2.0943951023817848  RotationAngleUnits=rad  RotationArbitraryAxis=[0 0 1]  RotationSequenceAxes=FollowerAxes  RotationSequence=XYX  RotationSequenceAngles=[0 0 0]  RotationSequenceAnglesUnits=deg  RotationMatrix=[1 0 0; 0 1 0; 0 0 1]  Quaternion=[1 0 0 0]  TranslationMethod=Cartesian  TranslationCartesianOffset=[99.809427786814155 172.87499999886114 24.000000000062251]  TranslationCartesianOffsetUnits=mm  TranslationStandardAxis=+Z  TranslationStandardOffset=0  TranslationStandardOffsetUnits=mm  TranslationROffset=0  TranslationROffsetUnits=m  TranslationThetaOffset=0  TranslationThetaOffsetUnits=deg  TranslationZOffset=0  TranslationZOffsetUnits=m
  Transform43 : sm_lib/Frames and Transforms/Rigid Transform  RotationMethod=ArbitraryAxis  FollAlignAxisA=+X  BaseAlignAxisA=+Y  FollAlignAxisB=+Y  BaseAlignAxisB=+Z  RotationStandardAxis=+Z  RotationAngle=2.0943951024046012  RotationAngleUnits=rad  RotationArbitraryAxis=[-0 -0 -1]  RotationSequenceAxes=FollowerAxes  RotationSequence=XYX  RotationSequenceAngles=[0 0 0]  RotationSequenceAnglesUnits=deg  RotationMatrix=[1 0 0; 0 1 0; 0 0 1]  Quaternion=[1 0 0 0]  TranslationMethod=Cartesian  TranslationCartesianOffset=[-99.809427785499309 172.87500000113846 24.000000000062251]  TranslationCartesianOffsetUnits=mm  TranslationStandardAxis=+Z  TranslationStandardOffset=0  TranslationStandardOffsetUnits=mm  TranslationROffset=0  TranslationROffsetUnits=m  TranslationThetaOffset=0  TranslationThetaOffsetUnits=deg  TranslationZOffset=0  TranslationZOffsetUnits=m
  Transform44 : sm_lib/Frames and Transforms/Rigid Transform  RotationMethod=ArbitraryAxis  FollAlignAxisA=+X  BaseAlignAxisA=+Y  FollAlignAxisB=+Y  BaseAlignAxisB=+Z  RotationStandardAxis=+Z  RotationAngle=1.5707963267948968  RotationAngleUnits=rad  RotationArbitraryAxis=[-0 -1 -0]  RotationSequenceAxes=FollowerAxes  RotationSequence=XYX  RotationSequenceAngles=[0 0 0]  RotationSequenceAnglesUnits=deg  RotationMatrix=[1 0 0; 0 1 0; 0 0 1]  Quaternion=[1 0 0 0]  TranslationMethod=Cartesian  TranslationCartesianOffset=[13.533207794599599 64.174992098843177 13.600000000000001]  TranslationCartesianOffsetUnits=mm  TranslationStandardAxis=+Z  TranslationStandardOffset=0  TranslationStandardOffsetUnits=mm  TranslationROffset=0  TranslationROffsetUnits=m  TranslationThetaOffset=0  TranslationThetaOffsetUnits=deg  TranslationZOffset=0  TranslationZOffsetUnits=m
  Transform45 : sm_lib/Frames and Transforms/Rigid Transform  RotationMethod=ArbitraryAxis  FollAlignAxisA=+X  BaseAlignAxisA=+Y  FollAlignAxisB=+Y  BaseAlignAxisB=+Z  RotationStandardAxis=+Z  RotationAngle=2.7572489937583149  RotationAngleUnits=rad  RotationArbitraryAxis=[-0.69359259312433763 -0.19457294140273607 -0.69359259312433874]  RotationSequenceAxes=FollowerAxes  RotationSequence=XYX  RotationSequenceAngles=[0 0 0]  RotationSequenceAnglesUnits=deg  RotationMatrix=[1 0 0; 0 1 0; 0 0 1]  Quaternion=[1 0 0 0]  TranslationMethod=Cartesian  TranslationCartesianOffset=[84.567755458442107 126.06222448336912 36.100000000000037]  TranslationCartesianOffsetUnits=mm  TranslationStandardAxis=+Z  TranslationStandardOffset=0  TranslationStandardOffsetUnits=mm  TranslationROffset=0  TranslationROffsetUnits=m  TranslationThetaOffset=0  TranslationThetaOffsetUnits=deg  TranslationZOffset=0  TranslationZOffsetUnits=m
  Transform46 : sm_lib/Frames and Transforms/Rigid Transform  RotationMethod=ArbitraryAxis  FollAlignAxisA=+X  BaseAlignAxisA=+Y  FollAlignAxisB=+Y  BaseAlignAxisB=+Z  RotationStandardAxis=+Z  RotationAngle=1.6320911114092145  RotationAngleUnits=rad  RotationArbitraryAxis=[-0.24025122409678262 -0.94050980783827787 -0.24025122409678393]  RotationSequenceAxes=FollowerAxes  RotationSequence=XYX  RotationSequenceAngles=[0 0 0]  RotationSequenceAnglesUnits=deg  RotationMatrix=[1 0 0; 0 1 0; 0 0 1]  Quaternion=[1 0 0 0]  TranslationMethod=Cartesian  TranslationCartesianOffset=[-51.647538803239108 183.08171232635618 36.100000000000037]  TranslationCartesianOffsetUnits=mm  TranslationStandardAxis=+Z  TranslationStandardOffset=0  TranslationStandardOffsetUnits=mm  TranslationROffset=0  TranslationROffsetUnits=m  TranslationThetaOffset=0  TranslationThetaOffsetUnits=deg  TranslationZOffset=0  TranslationZOffsetUnits=m
  Transform47 : sm_lib/Frames and Transforms/Rigid Transform  RotationMethod=ArbitraryAxis  FollAlignAxisA=+X  BaseAlignAxisA=+Y  FollAlignAxisB=+Y  BaseAlignAxisB=+Z  RotationStandardAxis=+Z  RotationAngle=3.1415926535897922  RotationAngleUnits=rad  RotationArbitraryAxis=[0.99207089132052606 -0.125679539283437 6.6259454489207254e-17]  RotationSequenceAxes=FollowerAxes  RotationSequence=XYX  RotationSequenceAngles=[0 0 0]  RotationSequenceAnglesUnits=deg  RotationMatrix=[1 0 0; 0 1 0; 0 0 1]  Quaternion=[1 0 0 0]  TranslationMethod=Cartesian  TranslationCartesianOffset=[67.670238338594061 154.67994478363838 38.499999999999979]  TranslationCartesianOffsetUnits=mm  TranslationStandardAxis=+Z  TranslationStandardOffset=0  TranslationStandardOffsetUnits=mm  TranslationROffset=0  TranslationROffsetUnits=m  TranslationThetaOffset=0  TranslationThetaOffsetUnits=deg  TranslationZOffset=0  TranslationZOffsetUnits=m
  Transform48 : sm_lib/Frames and Transforms/Rigid Transform  RotationMethod=ArbitraryAxis  FollAlignAxisA=+X  BaseAlignAxisA=+Y  FollAlignAxisB=+Y  BaseAlignAxisB=+Z  RotationStandardAxis=+Z  RotationAngle=3.1415926535897931  RotationAngleUnits=rad  RotationArbitraryAxis=[0.60487711941564182 0.79631882459692971 4.2817701064170949e-16]  RotationSequenceAxes=FollowerAxes  RotationSequence=XYX  RotationSequenceAngles=[0 0 0]  RotationSequenceAnglesUnits=deg  RotationMatrix=[1 0 0; 0 1 0; 0 0 1]  Quaternion=[1 0 0 0]  TranslationMethod=Cartesian  TranslationCartesianOffset=[-67.982453021745741 154.13917308955064 38.499999999999979]  TranslationCartesianOffsetUnits=mm  TranslationStandardAxis=+Z  TranslationStandardOffset=0  TranslationStandardOffsetUnits=mm  TranslationROffset=0  TranslationROffsetUnits=m  TranslationThetaOffset=0  TranslationThetaOffsetUnits=deg  TranslationZOffset=0  TranslationZOffsetUnits=m
  Transform49 : sm_lib/Frames and Transforms/Rigid Transform  RotationMethod=ArbitraryAxis  FollAlignAxisA=+X  BaseAlignAxisA=+Y  FollAlignAxisB=+Y  BaseAlignAxisB=+Z  RotationStandardAxis=+Z  RotationAngle=1.5865923302678127  RotationAngleUnits=rad  RotationArbitraryAxis=[-0.98432745245712761 0.12469856923650148 -0.12469856923650251]  RotationSequenceAxes=FollowerAxes  RotationSequence=XYX  RotationSequenceAngles=[0 0 0]  RotationSequenceAnglesUnits=deg  RotationMatrix=[1 0 0; 0 1 0; 0 0 1]  Quaternion=[1 0 0 0]  TranslationMethod=Cartesian  TranslationCartesianOffset=[53.955106957250102 101.41743290903302 38.500000000000028]  TranslationCartesianOffsetUnits=mm  TranslationStandardAxis=+Z  TranslationStandardOffset=0  TranslationStandardOffsetUnits=mm  TranslationROffset=0  TranslationROffsetUnits=m  TranslationThetaOffset=0  TranslationThetaOffsetUnits=deg  TranslationZOffset=0  TranslationZOffsetUnits=m
  Transform5 : sm_lib/Frames and Transforms/Rigid Transform  RotationMethod=ArbitraryAxis  FollAlignAxisA=+X  BaseAlignAxisA=+Y  FollAlignAxisB=+Y  BaseAlignAxisB=+Z  RotationStandardAxis=+Z  RotationAngle=2.4188584057763802  RotationAngleUnits=rad  RotationArbitraryAxis=[0.65465367070797764 -0.37796447300922548 0.65465367070797764]  RotationSequenceAxes=FollowerAxes  RotationSequence=XYX  RotationSequenceAngles=[0 0 0]  RotationSequenceAnglesUnits=deg  RotationMatrix=[1 0 0; 0 1 0; 0 0 1]  Quaternion=[1 0 0 0]  TranslationMethod=Cartesian  TranslationCartesianOffset=[38.79750556351344 129.92818230283672 49.100000000000001]  TranslationCartesianOffsetUnits=mm  TranslationStandardAxis=+Z  TranslationStandardOffset=0  TranslationStandardOffsetUnits=mm  TranslationROffset=0  TranslationROffsetUnits=m  TranslationThetaOffset=0  TranslationThetaOffsetUnits=deg  TranslationZOffset=0  TranslationZOffsetUnits=m
  Transform50 : sm_lib/Frames and Transforms/Rigid Transform  RotationMethod=ArbitraryAxis  FollAlignAxisA=+X  BaseAlignAxisA=+Y  FollAlignAxisB=+Y  BaseAlignAxisB=+Z  RotationStandardAxis=+Z  RotationAngle=2.2576709855630233  RotationAngleUnits=rad  RotationArbitraryAxis=[-0.47317816576134758 -0.62293756647304876 0.62293756647304777]  RotationSequenceAxes=FollowerAxes  RotationSequence=XYX  RotationSequenceAngles=[0 0 0]  RotationSequenceAnglesUnits=deg  RotationMatrix=[1 0 0; 0 1 0; 0 0 1]  Quaternion=[1 0 0 0]  TranslationMethod=Cartesian  TranslationCartesianOffset=[-14.998198978295296 168.8927768343685 38.500000000000028]  TranslationCartesianOffsetUnits=mm  TranslationStandardAxis=+Z  TranslationStandardOffset=0  TranslationStandardOffsetUnits=mm  TranslationROffset=0  TranslationROffsetUnits=m  TranslationThetaOffset=0  TranslationThetaOffsetUnits=deg  TranslationZOffset=0  TranslationZOffsetUnits=m
  Transform51 : sm_lib/Frames and Transforms/Rigid Transform  RotationMethod=ArbitraryAxis  FollAlignAxisA=+X  BaseAlignAxisA=+Y  FollAlignAxisB=+Y  BaseAlignAxisB=+Z  RotationStandardAxis=+Z  RotationAngle=2.4188584057763807  RotationAngleUnits=rad  RotationArbitraryAxis=[0.65465367070797775 -0.37796447300922559 0.65465367070797753]  RotationSequenceAxes=FollowerAxes  RotationSequence=XYX  RotationSequenceAngles=[0 0 0]  RotationSequenceAnglesUnits=deg  RotationMatrix=[1 0 0; 0 1 0; 0 0 1]  Quaternion=[1 0 0 0]  TranslationMethod=Cartesian  TranslationCartesianOffset=[37.465650443592779 152.50760569539543 13.600000000000001]  TranslationCartesianOffsetUnits=mm  TranslationStandardAxis=+Z  TranslationStandardOffset=0  TranslationStandardOffsetUnits=mm  TranslationROffset=0  TranslationROffsetUnits=m  TranslationThetaOffset=0  TranslationThetaOffsetUnits=deg  TranslationZOffset=0  TranslationZOffsetUnits=m
  Transform52 : sm_lib/Frames and Transforms/Rigid Transform  RotationMethod=ArbitraryAxis  FollAlignAxisA=+X  BaseAlignAxisA=+Y  FollAlignAxisB=+Y  BaseAlignAxisB=+Z  RotationStandardAxis=+Z  RotationAngle=2.4188584057763718  RotationAngleUnits=rad  RotationArbitraryAxis=[-0.6546536707079762 -0.37796447300923069 -0.65465367070797598]  RotationSequenceAxes=FollowerAxes  RotationSequence=XYX  RotationSequenceAngles=[0 0 0]  RotationSequenceAnglesUnits=deg  RotationMatrix=[1 0 0; 0 1 0; 0 0 1]  Quaternion=[1 0 0 0]  TranslationMethod=Cartesian  TranslationCartesianOffset=[-50.998858238192668 129.06740220576114 13.600000000000001]  TranslationCartesianOffsetUnits=mm  TranslationStandardAxis=+Z  TranslationStandardOffset=0  TranslationStandardOffsetUnits=mm  TranslationROffset=0  TranslationROffsetUnits=m  TranslationThetaOffset=0  TranslationThetaOffsetUnits=deg  TranslationZOffset=0  TranslationZOffsetUnits=m
  Transform53 : sm_lib/Frames and Transforms/Rigid Transform  RotationMethod=None  FollAlignAxisA=+X  BaseAlignAxisA=+Y  FollAlignAxisB=+Y  BaseAlignAxisB=+Z  RotationStandardAxis=+Z  RotationAngle=0  RotationAngleUnits=deg  RotationArbitraryAxis=[0 0 1]  RotationSequenceAxes=FollowerAxes  RotationSequence=XYX  RotationSequenceAngles=[0 0 0]  RotationSequenceAnglesUnits=deg  RotationMatrix=[1 0 0; 0 1 0; 0 0 1]  Quaternion=[1 0 0 0]  TranslationMethod=None  TranslationCartesianOffset=[0 0 0]  TranslationCartesianOffsetUnits=m  TranslationStandardAxis=+Z  TranslationStandardOffset=0  TranslationStandardOffsetUnits=m  TranslationROffset=0  TranslationROffsetUnits=m  TranslationThetaOffset=0  TranslationThetaOffsetUnits=deg  TranslationZOffset=0  TranslationZOffsetUnits=m
  Transform54 : sm_lib/Frames and Transforms/Rigid Transform  RotationMethod=None  FollAlignAxisA=+X  BaseAlignAxisA=+Y  FollAlignAxisB=+Y  BaseAlignAxisB=+Z  RotationStandardAxis=+Z  RotationAngle=0  RotationAngleUnits=rad  RotationArbitraryAxis=[1 0 0]  RotationSequenceAxes=FollowerAxes  RotationSequence=XYX  RotationSequenceAngles=[0 0 0]  RotationSequenceAnglesUnits=deg  RotationMatrix=[1 0 0; 0 1 0; 0 0 1]  Quaternion=[1 0 0 0]  TranslationMethod=Cartesian  TranslationCartesianOffset=[-30 40 75]  TranslationCartesianOffsetUnits=mm  TranslationStandardAxis=+Z  TranslationStandardOffset=200  TranslationStandardOffsetUnits=mm  TranslationROffset=0  TranslationROffsetUnits=m  TranslationThetaOffset=0  TranslationThetaOffsetUnits=deg  TranslationZOffset=0  TranslationZOffsetUnits=m
  Transform6 : sm_lib/Frames and Transforms/Rigid Transform  RotationMethod=ArbitraryAxis  FollAlignAxisA=+X  BaseAlignAxisA=+Y  FollAlignAxisB=+Y  BaseAlignAxisB=+Z  RotationStandardAxis=+Z  RotationAngle=3.1415926535897931  RotationAngleUnits=rad  RotationArbitraryAxis=[0.98901586336191671 0.14780941112961193 -7.4147043167175484e-17]  RotationSequenceAxes=FollowerAxes  RotationSequence=XYX  RotationSequenceAngles=[0 0 0]  RotationSequenceAnglesUnits=deg  RotationMatrix=[1 0 0; 0 1 0; 0 0 1]  Quaternion=[1 0 0 0]  TranslationMethod=Cartesian  TranslationCartesianOffset=[10.619396930206873 115.03911940923673 52.900000000000013]  TranslationCartesianOffsetUnits=mm  TranslationStandardAxis=+Z  TranslationStandardOffset=0  TranslationStandardOffsetUnits=mm  TranslationROffset=0  TranslationROffsetUnits=m  TranslationThetaOffset=0  TranslationThetaOffsetUnits=deg  TranslationZOffset=0  TranslationZOffsetUnits=m
  Transform7 : sm_lib/Frames and Transforms/Rigid Transform  RotationMethod=ArbitraryAxis  FollAlignAxisA=+X  BaseAlignAxisA=+Y  FollAlignAxisB=+Y  BaseAlignAxisB=+Z  RotationStandardAxis=+Z  RotationAngle=3.1415926535897927  RotationAngleUnits=rad  RotationArbitraryAxis=[0.38719377190488019 -0.92199836388036582 -3.5277797665665267e-16]  RotationSequenceAxes=FollowerAxes  RotationSequence=XYX  RotationSequenceAngles=[0 0 0]  RotationSequenceAnglesUnits=deg  RotationMatrix=[1 0 0; 0 1 0; 0 0 1]  Quaternion=[1 0 0 0]  TranslationMethod=Cartesian  TranslationCartesianOffset=[0.3122146831511497 36.930882126810701 38.499999999999979]  TranslationCartesianOffsetUnits=mm  TranslationStandardAxis=+Z  TranslationStandardOffset=0  TranslationStandardOffsetUnits=mm  TranslationROffset=0  TranslationROffsetUnits=m  TranslationThetaOffset=0  TranslationThetaOffsetUnits=deg  TranslationZOffset=0  TranslationZOffsetUnits=m
  Transform8 : sm_lib/Frames and Transforms/Rigid Transform  RotationMethod=ArbitraryAxis  FollAlignAxisA=+X  BaseAlignAxisA=+Y  FollAlignAxisB=+Y  BaseAlignAxisB=+Z  RotationStandardAxis=+Z  RotationAngle=3.1415926535897931  RotationAngleUnits=rad  RotationArbitraryAxis=[0.36650122672429392 0.93041756798202591 2.9831310769236364e-17]  RotationSequenceAxes=FollowerAxes  RotationSequence=XYX  RotationSequenceAngles=[0 0 0]  RotationSequenceAnglesUnits=deg  RotationMatrix=[1 0 0; 0 1 0; 0 0 1]  Quaternion=[1 0 0 0]  TranslationMethod=Cartesian  TranslationCartesianOffset=[-5.1270705163374286 124.55210780981125 52.900000000000013]  TranslationCartesianOffsetUnits=mm  TranslationStandardAxis=+Z  TranslationStandardOffset=0  TranslationStandardOffsetUnits=mm  TranslationROffset=0  TranslationROffsetUnits=m  TranslationThetaOffset=0  TranslationThetaOffsetUnits=deg  TranslationZOffset=0  TranslationZOffsetUnits=m
  Transform9 : sm_lib/Frames and Transforms/Rigid Transform  RotationMethod=ArbitraryAxis  FollAlignAxisA=+X  BaseAlignAxisA=+Y  FollAlignAxisB=+Y  BaseAlignAxisB=+Z  RotationStandardAxis=+Z  RotationAngle=1.6198107529808947  RotationAngleUnits=rad  RotationArbitraryAxis=[0.21611670615757558 -0.95214869565588378 0.21611670615757447]  RotationSequenceAxes=FollowerAxes  RotationSequence=XYX  RotationSequenceAngles=[0 0 0]  RotationSequenceAnglesUnits=deg  RotationMatrix=[1 0 0; 0 1 0; 0 0 1]  Quaternion=[1 0 0 0]  TranslationMethod=Cartesian  TranslationCartesianOffset=[-39.03991378494019 137.80425887104397 36.099999999999966]  TranslationCartesianOffsetUnits=mm  TranslationStandardAxis=+Z  TranslationStandardOffset=0  TranslationStandardOffsetUnits=mm  TranslationROffset=0  TranslationROffsetUnits=m  TranslationThetaOffset=0  TranslationThetaOffsetUnits=deg  TranslationZOffset=0  TranslationZOffsetUnits=m
  Vis_tle_tte_cylindrique_cruciforme_H_29x13_C_10_RIGID : Subsystem
  Vis_tle_tte_cylindrique_cruciforme_H_29x13_C_11_RIGID : Subsystem
  Vis_tle_tte_cylindrique_cruciforme_H_29x13_C_12_RIGID : Subsystem
  Vis_tle_tte_cylindrique_cruciforme_H_29x13_C_13_RIGID : Subsystem
  Vis_tle_tte_cylindrique_cruciforme_H_29x13_C_14_RIGID : Subsystem
  Vis_tle_tte_cylindrique_cruciforme_H_29x13_C_15_RIGID : Subsystem
  Vis_tle_tte_cylindrique_cruciforme_H_29x13_C_16_RIGID : Subsystem
  Vis_tle_tte_cylindrique_cruciforme_H_29x13_C_17_RIGID : Subsystem
  Vis_tle_tte_cylindrique_cruciforme_H_29x13_C_18_RIGID : Subsystem
  Vis_tle_tte_cylindrique_cruciforme_H_29x13_C_19_RIGID : Subsystem
  Vis_tle_tte_cylindrique_cruciforme_H_29x13_C_1_RIGID : Subsystem
  Vis_tle_tte_cylindrique_cruciforme_H_29x13_C_20_RIGID : Subsystem
  Vis_tle_tte_cylindrique_cruciforme_H_29x13_C_21_RIGID : Subsystem
  Vis_tle_tte_cylindrique_cruciforme_H_29x13_C_22_RIGID : Subsystem
  Vis_tle_tte_cylindrique_cruciforme_H_29x13_C_23_RIGID : Subsystem
  Vis_tle_tte_cylindrique_cruciforme_H_29x13_C_2_RIGID : Subsystem
  Vis_tle_tte_cylindrique_cruciforme_H_29x13_C_3_RIGID : Subsystem
  Vis_tle_tte_cylindrique_cruciforme_H_29x13_C_4_RIGID : Subsystem
  Vis_tle_tte_cylindrique_cruciforme_H_29x13_C_5_RIGID : Subsystem
  Vis_tle_tte_cylindrique_cruciforme_H_29x13_C_7_RIGID : Subsystem
  Vis_tle_tte_cylindrique_cruciforme_H_29x13_C_8_RIGID : Subsystem
  Vis_tle_tte_cylindrique_cruciforme_H_29x13_C_9_RIGID : Subsystem
  Vis_tle_tte_cylindrique_cruciforme_H_29x8_C_1_RIGID : Subsystem
  Vis_tle_tte_cylindrique_cruciforme_H_29x8_C_2_RIGID : Subsystem
  Vis_tle_tte_cylindrique_cruciforme_H_29x8_C_3_RIGID : Subsystem
  carter_avant_1_RIGID : Subsystem
  carter_transparant_5_RIGID : Subsystem
  petite_carte_1_RIGID : Subsystem
  petite_carte_2_RIGID : Subsystem
  petite_carte_3_RIGID : Subsystem
  plaque_fixation_1_RIGID : Subsystem
  socle_1_RIGID : Subsystem
  vis_CHC_M4_30_1_RIGID : Subsystem
  vis_CHC_M4_30_2_RIGID : Subsystem
  F5 : PMIOPort  Side=Left
  F4 : PMIOPort  Port=2  Side=Right
  F3 : PMIOPort  Port=3  Side=Right
  F2 : PMIOPort  Port=4  Side=Right
  F1 : PMIOPort  Port=5  Side=Right
  F : PMIOPort  Port=6  Side=Right
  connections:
  Transform/LConn1 -- Transform54/LConn1 -- Transform8/LConn1 -- Transform9/LConn1 -- Transform7/LConn1 -- Transform6/LConn1 -- Transform53/LConn1 -- Transform52/LConn1 -- Transform51/LConn1 -- Transform50/LConn1 -- Transform5/LConn1 -- Transform49/LConn1 -- Transform48/LConn1 -- Transform47/LConn1 -- Transform46/LConn1 -- Transform45/LConn1 -- Transform44/LConn1 -- Transform43/LConn1 -- Transform42/LConn1 -- Transform41/LConn1 -- Transform40/LConn1 -- Transform4/LConn1 -- Transform39/LConn1 -- Transform38/LConn1 -- Transform37/LConn1 -- Transform36/LConn1 -- Transform35/LConn1 -- Transform34/LConn1 -- ReferenceFrame/RConn1 -- carter_avant_1_RIGID/RConn1 -- carter_transparant_5_RIGID/RConn1 -- F5/RConn1 -- Transform33/LConn1 -- Transform32/LConn1 -- Transform31/LConn1 -- Transform30/LConn1 -- Transform3/LConn1 -- Transform29/LConn1 -- Transform28/LConn1 -- Transform27/LConn1 -- Transform26/LConn1 -- Transform25/LConn1 -- Transform24/LConn1 -- Transform23/LConn1 -- Transform22/LConn1 -- Transform21/LConn1 -- Transform20/LConn1 -- Transform2/LConn1 -- Transform19/LConn1 -- Transform18/LConn1 -- Transform17/LConn1 -- Transform16/LConn1 -- Transform15/LConn1 -- Transform14/LConn1 -- Transform13/LConn1 -- Transform12/LConn1 -- Transform11/LConn1 -- Transform10/LConn1 -- Transform1/LConn1
  Transform/RConn1 -- F/RConn1
  Transform9/RConn1 -- Vis_tle_tte_cylindrique_cruciforme_H_29x13_C_11_RIGID/LConn1
  Transform10/RConn1 -- Vis_tle_tte_cylindrique_cruciforme_H_29x13_C_13_RIGID/LConn1
  Transform11/RConn1 -- Vis_tle_tte_cylindrique_cruciforme_H_29x13_C_9_RIGID/LConn1
  Transform12/RConn1 -- Vis_tle_tte_cylindrique_cruciforme_H_29x13_C_8_RIGID/LConn1
  Transform13/RConn1 -- Vis_tle_tte_cylindrique_cruciforme_H_29x8_C_3_RIGID/LConn1
  Transform14/RConn1 -- Vis_tle_tte_cylindrique_cruciforme_H_29x13_C_12_RIGID/LConn1
  Transform15/RConn1 -- Vis_tle_tte_cylindrique_cruciforme_H_29x13_C_10_RIGID/LConn1
  Rondelle_M4_2_RIGID/LConn1 -- Transform16/RConn1
  CARTE_HEXAGONALE_1_RIGID/LConn1 -- Transform17/RConn1
  Transform18/RConn1 -- Vis_tle_tte_cylindrique_cruciforme_H_29x13_C_5_RIGID/LConn1
  Transform1/RConn1 -- F1/RConn1
  Transform19/RConn1 -- petite_carte_1_RIGID/LConn1
  Transform20/RConn1 -- Vis_tle_tte_cylindrique_cruciforme_H_29x8_C_1_RIGID/LConn1
  FIXATION_MOTEUR_1_RIGID/LConn1 -- Transform21/RConn1
  FIXATION_MOTEUR_2_RIGID/LConn1 -- Transform22/RConn1
  Transform23/RConn1 -- Vis_tle_tte_cylindrique_cruciforme_H_29x13_C_1_RIGID/LConn1
  Transform24/RConn1 -- Vis_tle_tte_cylindrique_cruciforme_H_29x13_C_2_RIGID/LConn1
  Transform25/RConn1 -- Vis_tle_tte_cylindrique_cruciforme_H_29x13_C_3_RIGID/LConn1
  Transform26/RConn1 -- Vis_tle_tte_cylindrique_cruciforme_H_29x13_C_4_RIGID/LConn1
  Transform27/RConn1 -- socle_1_RIGID/LConn1
  Transform28/RConn1 -- vis_CHC_M4_30_1_RIGID/LConn1
  Transform2/RConn1 -- F2/RConn1
  Transform29/RConn1 -- vis_CHC_M4_30_2_RIGID/LConn1
  Rondelle_M4_1_RIGID/LConn1 -- Transform30/RConn1
  CARTER_ARRIERE_1_RIGID/LConn1 -- Transform31/RConn1
  Transform32/RConn1 -- Vis_tle_tte_cylindrique_cruciforme_H_29x13_C_18_RIGID/LConn1
  Transform33/RConn1 -- Vis_tle_tte_cylindrique_cruciforme_H_29x13_C_19_RIGID/LConn1
  Transform34/RConn1 -- Vis_tle_tte_cylindrique_cruciforme_H_29x13_C_20_RIGID/LConn1
  Transform35/RConn1 -- Vis_tle_tte_cylindrique_cruciforme_H_29x13_C_21_RIGID/LConn1
  Transform36/RConn1 -- Vis_tle_tte_cylindrique_cruciforme_H_29x13_C_22_RIGID/LConn1
  Transform37/RConn1 -- Vis_tle_tte_cylindrique_cruciforme_H_29x13_C_23_RIGID/LConn1
  FIXATION_MOTEUR_5_RIGID/LConn1 -- Transform38/RConn1
  Transform3/RConn1 -- F3/RConn1
  FIXATION_MOTEUR_6_RIGID/LConn1 -- Transform39/RConn1
  PLAQUE_NOM_1_RIGID/LConn1 -- Transform40/RConn1
  CACHE_1_RIGID/LConn1 -- Transform41/RConn1
  CACHE_2_RIGID/LConn1 -- Transform42/RConn1
  CACHE_3_RIGID/LConn1 -- Transform43/RConn1
  Transform44/RConn1 -- Vis_tle_tte_cylindrique_cruciforme_H_29x13_C_7_RIGID/LConn1
  Transform45/RConn1 -- Vis_tle_tte_cylindrique_cruciforme_H_29x13_C_14_RIGID/LConn1
  Transform46/RConn1 -- Vis_tle_tte_cylindrique_cruciforme_H_29x13_C_15_RIGID/LConn1
  MOTEUR_2_RIGID/LConn1 -- Transform47/RConn1
  MOTEUR_3_RIGID/LConn1 -- Transform48/RConn1
  Transform4/RConn1 -- F4/RConn1
  FIXATION_MOTEUR_3_RIGID/LConn1 -- Transform49/RConn1
  FIXATION_MOTEUR_4_RIGID/LConn1 -- Transform50/RConn1
  Transform51/RConn1 -- Vis_tle_tte_cylindrique_cruciforme_H_29x13_C_16_RIGID/LConn1
  Transform52/RConn1 -- Vis_tle_tte_cylindrique_cruciforme_H_29x13_C_17_RIGID/LConn1
  Transform53/RConn1 -- plaque_fixation_1_RIGID/LConn1
  Transform5/RConn1 -- Vis_tle_tte_cylindrique_cruciforme_H_29x8_C_2_RIGID/LConn1
  Transform6/RConn1 -- petite_carte_2_RIGID/LConn1
  MOTEUR_1_RIGID/LConn1 -- Transform7/RConn1
  Transform8/RConn1 -- petite_carte_3_RIGID/LConn1
  PLAQUE_NOM_SET/LConn1 -- Transform54/RConn1
